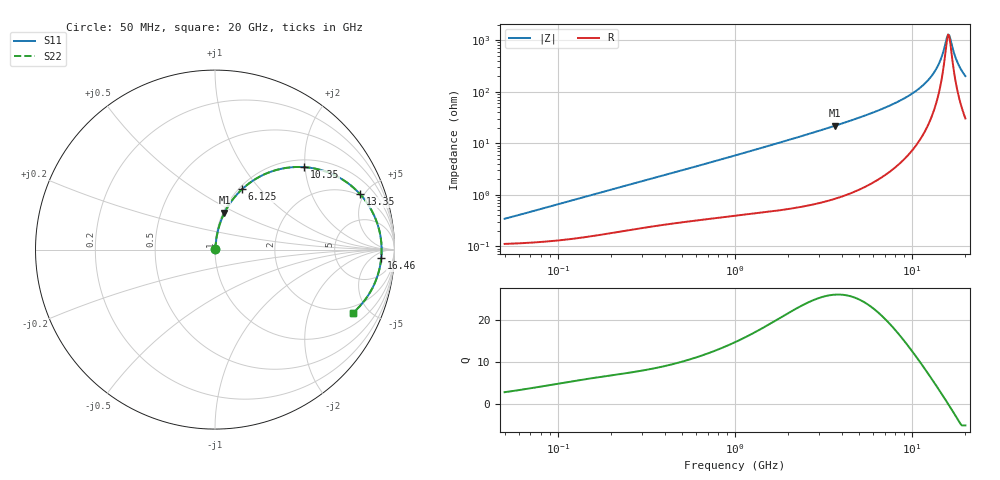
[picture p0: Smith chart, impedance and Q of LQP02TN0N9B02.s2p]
!Murata Part Number: LQP02TN0N9B02
!These Parameters are Measured in Series Mode Connection
!  o--[Z]--o
!Port1  Port2
!  o-------o
!Freq. Start=50[MHz] Stop=20[GHz], 401[Steps]
# Hz S RI R 50
!Freq.(Hz) S11(Real) S11(Imag) S21(Real) S21(Imag) S12(Real) S12(Imag) S22(Real) S22(Imag)
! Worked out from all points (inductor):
!   401 points, 50 MHz to 20 GHz, reference 50 ohm
!   read as one part in series: L = 1.03 nH near 52.3 MHz
!   highest Q = 26.1 at 3.681 GHz (marker M1), where L = 946 pH
!   self-resonance near 16.05 GHz
!   S11 on the Smith chart (normalised r, x): 50 MHz: 1.00, +0.01; 6.125 GHz: 1.04, +0.81; 10.35 GHz: 1.17, +1.98; 13.35 GHz: 1.91, +4.69; 16.46 GHz: 18, -12; 20 GHz: 1.60, -3.97
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5e7  0.00112 0.00323  0.9989 -0.00323  0.9989 -0.00323  0.00112 0.00323
1.364002e8  0.00155 0.00863  0.9985 -0.00863  0.9985 -0.00863  0.00155 0.00863
3.721004e8  0.00302 0.0222  0.997 -0.0222  0.997 -0.0222  0.00302 0.0222
1e9  0.00716 0.057  0.9928 -0.057  0.9928 -0.057  0.00716 0.057
2.728004e9  0.0304 0.1527  0.9696 -0.1527  0.9696 -0.1527  0.0304 0.1527
3.680849e9  0.0529 0.2054  0.9471 -0.2054  0.9471 -0.2054  0.0529 0.2054
6.125241e9  0.1504 0.3361  0.8496 -0.3361  0.8496 -0.3361  0.1504 0.3361
7.442007e9  0.2324 0.3972  0.7676 -0.3972  0.7676 -0.3972  0.2324 0.3972
8.774992e9  0.34 0.443  0.66 -0.443  0.66 -0.443  0.34 0.443
1.034674e10  0.4964 0.4595  0.5036 -0.4595  0.5036 -0.4595  0.4964 0.4595
1.201863e10  0.6794 0.4082  0.3206 -0.4082  0.3206 -0.4082  0.6794 0.4082
1.334722e10  0.8092 0.3078  0.1908 -0.3078  0.1908 -0.3078  0.8092 0.3078
1.438523e10  0.8826 0.1987  0.1174 -0.1987  0.1174 -0.1987  0.8826 0.1987
1.482269e10  0.9036 0.1475  0.0964 -0.1475  0.0964 -0.1475  0.9036 0.1475
1.573793e10  0.9268 0.037  0.0732 -0.037  0.0732 -0.037  0.9268 0.037
1.597544e10  0.9284 0.00841  0.0716 -0.00841  0.0716 -0.00841  0.9284 0.00841
1.621653e10  0.9281 -0.0202  0.0719 0.0202  0.0719 0.0202  0.9281 -0.0202
1.646126e10  0.9261 -0.0488  0.0739 0.0488  0.0739 0.0488  0.9261 -0.0488
1.747767e10  0.9012 -0.1589  0.0988 0.1589  0.0988 0.1589  0.9012 -0.1589
1.800918e10  0.8795 -0.2097  0.1205 0.2097  0.1205 0.2097  0.8795 -0.2097
1.912117e10  0.8214 -0.2986  0.1786 0.2986  0.1786 0.2986  0.8214 -0.2986
2e10  0.7688 -0.3522  0.2312 0.3522  0.2312 0.3522  0.7688 -0.3522
